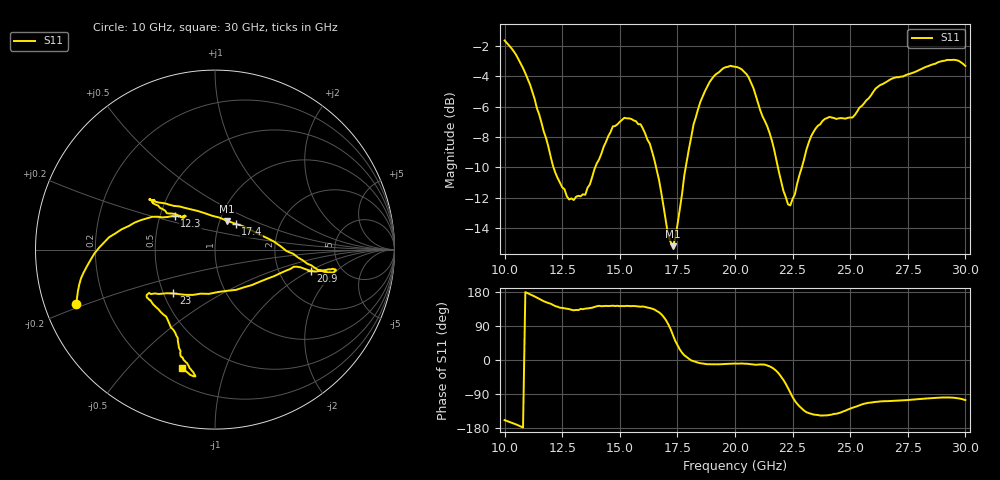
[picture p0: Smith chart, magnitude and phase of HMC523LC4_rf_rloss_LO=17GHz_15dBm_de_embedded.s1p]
!Hittite Microwave Corporation
!20 Alpha Rd
!Chelmsford, MA 01824
!Tel: 978-250-3343
!Fax: 978-250-3373
!Device: HMC523LC4, 10-30 GHz, GaAs MMIC Double-Balanced Mixer
!Misc: RF Return Loss with LO=17GHz at 15 dBm, Room
# MHZ S MA R 50
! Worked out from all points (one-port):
!   201 points, 10 GHz to 30 GHz, reference 50 ohm
!   lowest |S11| = -15.2 dB at 17.3 GHz (marker M1), VSWR 1.42, Z = 54.2 + j17.9 ohm
!   |S11| at or under -10 dB: 12.12 GHz to 13.93 GHz (1.808 GHz wide, 13.9 % of centre); 16.58 GHz to 17.86 GHz (1.281 GHz wide, 7.44 % of centre); 21.86 GHz to 22.9 GHz (1.038 GHz wide, 4.64 % of centre)
!   S11 on the Smith chart (normalised r, x): 10 GHz: 0.10, -0.19; 12.3 GHz: 0.60, +0.24; 17.4 GHz: 1.20, +0.36; 20.9 GHz: 3.02, -1.02; 23 GHz: 0.56, -0.31; 30 GHz: 0.29, -0.71
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10000  0.829 -158.7
10600  0.719 -172.7
11300  0.533 167.8
12300  0.292 140.6
12500  0.272 137.4
13500  0.257 135.6
15000  0.447 142.0
15700  0.449 142.1
16300  0.379 137.2
17300  0.174 67.0
17400  0.184 51.4
17500  0.204 39.5
18000  0.364 3.2
18500  0.521 -8.7
19100  0.634 -11.4
20000  0.679 -9.3
20500  0.642 -9.8
20900  0.546 -12.6
21700  0.362 -24.0
22300  0.239 -74.0
22500  0.249 -97.9
23000  0.337 -133.6
23900  0.457 -146.4
25000  0.462 -128.4
26100  0.575 -110.6
27500  0.641 -105.6
29200  0.715 -98.8
30000  0.683 -105.8
